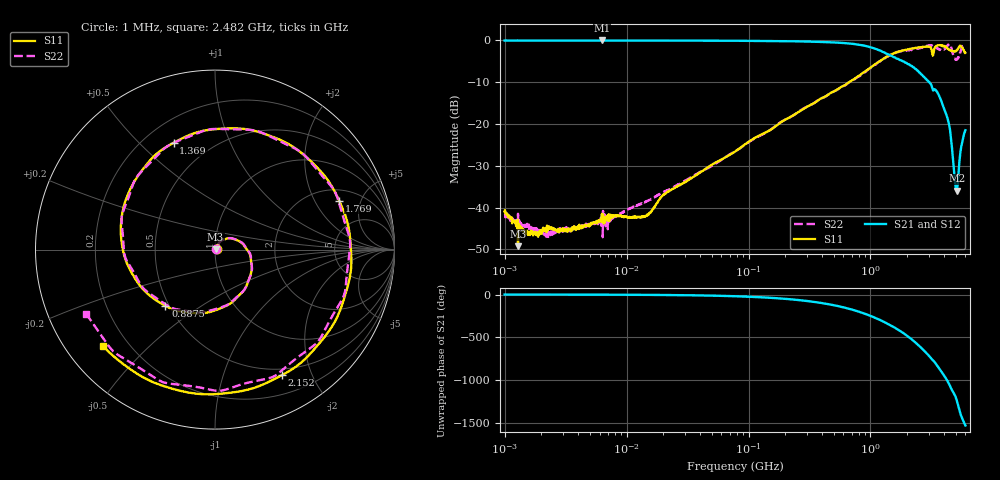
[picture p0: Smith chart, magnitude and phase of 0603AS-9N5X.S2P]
!s-Parameter Generated by FASTRON Sdn. Bhd.
!FASTRON P/N : 0603AS-9N5X
!Keysight Technologies: E5071C_MY46733604_B.14.02
!Date: Mon Dec 04 09:30:28 2023
!Version  :Rev01  Mon Dec 04 09:30:28 2023
!Data & Calibration Information:
!Freq  S11:SOLT2(ON)  S21:SOLT2(ON)  S12:SOLT2(ON)  S22:SOLT2(ON)
!PortZ  Port1:50+j0  Port2:50+j0
!When reading reference impedance value at option line is always used.
! Remarks : This data is being provided solely for informational purposes.
# Hz S dB R 50
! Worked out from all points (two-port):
!   1601 points, 1 MHz to 6 GHz, reference 50 ohm
!   highest |S21| = -0.03 dB at 6.282 MHz (marker M1); lowest = -36.0 dB at 5.105 GHz (marker M2)
!   |S21| within 3 dB of the highest: start of sweep to 1.32 GHz
!   lowest |S11| = -49.2 dB at 1.288 MHz (marker M3), VSWR 1.01, Z = 50.3 + j0.0883 ohm
!   |S11| at or under -10 dB: start of sweep to 668.3 MHz
!   |S22| runs from -47.1 to -0.8 dB; largest |S21 - S12| = 0.009
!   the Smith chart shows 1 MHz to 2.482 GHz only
!   S11 on the Smith chart (normalised r, x): 1 MHz: 1.02, +0.01; 887.5 MHz: 0.48, -0.36; 1.369 GHz: 0.32, +0.64; 1.769 GHz: 2.63, +3.22; 2.152 GHz: 0.42, -1.58; 2.482 GHz: 0.11, -0.37
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1000000  -40.91 21.6  -0.05 -0.1  -0.06 -0.2  -41.52 20.6
1287650  -49.23 14.7  -0.07 -0.1  -0.04 -0.2  -41.49 6.6
4277066  -44.93 37.2  -0.06 -1.1  -0.05 -1.1  -44.78 37.0
6281936  -41.48 49.4  -0.03 -1.8  -0.08 -1.3  -41.69 81.5
1.823719e7  -38.39 59.0  -0.06 -4.7  -0.07 -4.7  -36.95 56.2
7.757876e7  -26.60 58.6  -0.10 -19.7  -0.11 -19.7  -26.55 58.0
3.307917e8  -15.29 3.1  -0.31 -82.8  -0.31 -82.8  -15.34 4.5
6.317636e8  -10.52 -67.4  -0.69 -157.8  -0.69 -157.8  -10.60 -67.7
8.87456e8  -7.58 -131.4  -1.26 138.3  -1.26 138.3  -7.73 -131.2
1.368543e9  -3.90 111.2  -3.24 21.6  -3.24 21.7  -3.91 111.4
1.414819e9  -3.64 100.9  -3.44 10.5  -3.44 10.5  -3.70 99.3
1.769228e9  -2.57 21.5  -4.75 -70.2  -4.75 -70.2  -2.66 18.5
2.151902e9  -2.02 -62.1  -6.05 -158.7  -6.05 -158.5  -2.32 -72.7
2.482341e9  -1.70 -139.0  -7.53 123.8  -7.51 124.0  -1.91 -153.4
3.024401e9  -1.54 92.3  -9.95 1.5  -9.91 1.4  -1.31 90.5
3.361223e9  -1.78 31.4  -11.76 -72.6  -11.73 -72.8  -1.42 7.2
3.705459e9  -1.20 -48.5  -13.64 -156.8  -13.62 -157.0  -2.31 -82.2
4.19144e9  -1.75 -177.5  -17.81 89.2  -17.84 88.9  -1.66 174.4
4.545048e9  -2.46 84.0  -22.72 -7.1  -22.75 -7.2  -1.25 104.3
5.104645e9  -2.39 -30.8  -35.96 -162.8  -36.00 -162.5  -4.54 12.2
5.552322e9  -1.47 -111.0  -25.31 15.3  -25.33 15.6  -2.28 -99.0
6e9  -2.99 169.7  -21.50 -92.5  -21.51 -92.2  -0.93 158.1
